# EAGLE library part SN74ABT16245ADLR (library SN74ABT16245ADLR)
Texas Instruments SN74ABT16245ADLR, Dual, Bus Transceiver, 16-Bit Non-Inverting TTL, 5V, 48-Pin SSOP Source: Datasheet
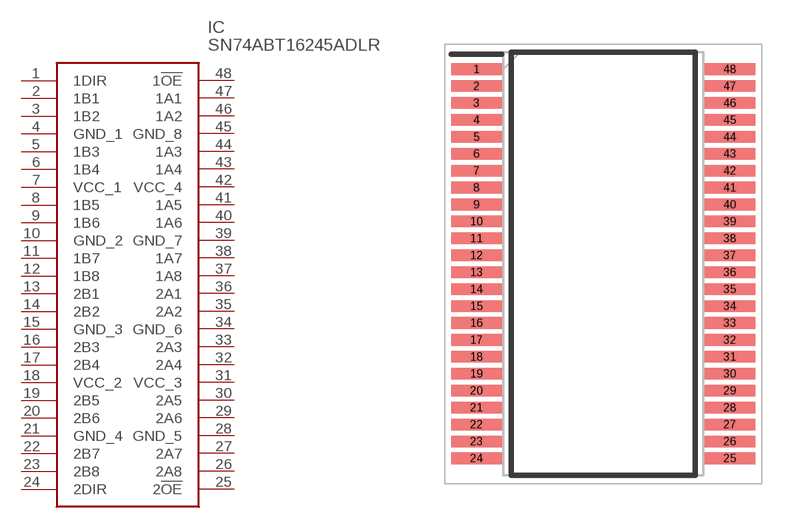
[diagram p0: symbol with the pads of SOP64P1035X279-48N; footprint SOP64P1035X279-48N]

Designator prefix IC

## SN74ABT16245ADLR (Description: Texas Instruments SN74ABT16245ADLR, Dual, Bus Transceiver, 16-Bit Non-Inverting TTL, 5V, 48-Pin SSOP; Height: 2.79mm; Manufacturer_Name: Texas Instruments; Manufacturer_Part_Number: SN74ABT16245ADLR; Mouser_Part_Number: 595-SN74ABT16245ADLR; Mouser_Price-Stock: https://www.mouser.co.uk/ProductDetail/Texas-Instruments/SN74ABT16245ADLR?qs=vxEfx8VrU7BbFiTJWgbLWw%3D%3D)  [SOP64P1035X279-48N]
1  1DIR
2  1B1
3  1B2
4  GND_1
5  1B3
6  1B4
7  VCC_1
8  1B5
9  1B6
10  GND_2
11  1B7
12  1B8
13  2B1
14  2B2
15  GND_3
16  2B3
17  2B4
18  VCC_2
19  2B5
20  2B6
21  GND_4
22  2B7
23  2B8
24  2DIR
25  2!OE
26  2A8
27  2A7
28  GND_5
29  2A6
30  2A5
31  VCC_3
32  2A4
33  2A3
34  GND_6
35  2A2
36  2A1
37  1A8
38  1A7
39  GND_7
40  1A6
41  1A5
42  VCC_4
43  1A4
44  1A3
45  GND_8
46  1A2
47  1A1
48  1!OE

## Footprint SOP64P1035X279-48N (pad centres in mm)
DL (R-PDSO-G48)
smd 1.9 x 0.435: 1 -4.75,7.302; 2 -4.75,6.668; 3 -4.75,6.032; 4 -4.75,5.398; 5 -4.75,4.762; 6 -4.75,4.128; 7 -4.75,3.492; 8 -4.75,2.858; 9 -4.75,2.222; 10 -4.75,1.588; 11 -4.75,0.952; 12 -4.75,0.318; 13 -4.75,-0.318; 14 -4.75,-0.952; 15 -4.75,-1.588; 16 -4.75,-2.222; 17 -4.75,-2.858; 18 -4.75,-3.492; 19 -4.75,-4.128; 20 -4.75,-4.762; 21 -4.75,-5.398; 22 -4.75,-6.032; 23 -4.75,-6.668; 24 -4.75,-7.302; 25 4.75,-7.302; 26 4.75,-6.668; 27 4.75,-6.032; 28 4.75,-5.398; 29 4.75,-4.762; 30 4.75,-4.128; 31 4.75,-3.492; 32 4.75,-2.858; 33 4.75,-2.222; 34 4.75,-1.588; 35 4.75,-0.952; 36 4.75,-0.318; 37 4.75,0.318; 38 4.75,0.952; 39 4.75,1.588; 40 4.75,2.222; 41 4.75,2.858; 42 4.75,3.492; 43 4.75,4.128; 44 4.75,4.762; 45 4.75,5.398; 46 4.75,6.032; 47 4.75,6.668; 48 4.75,7.302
